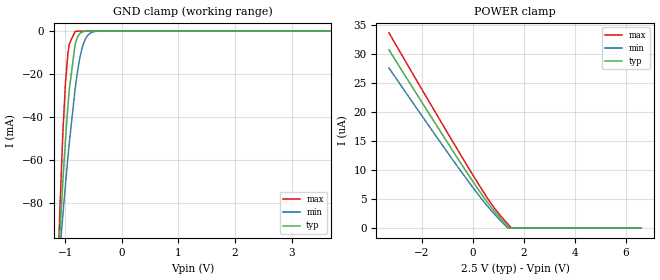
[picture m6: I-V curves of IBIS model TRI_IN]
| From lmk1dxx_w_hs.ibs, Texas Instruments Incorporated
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|   TRI_IN Model
[Model]   TRI_IN
Model_type   Input
Vinl = 0.75
Vinh = 1.75
|   typ   min   max
C_comp   1.93pF   1.8pF   2.08pF
[Voltage Range]   2.5   2.375   2.625
[Temperature Range]   45   150   -40
[Power Clamp Reference]   2.5   2.375   2.625
[GND Clamp Reference]   0   0   0
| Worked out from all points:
|   GND clamp passes 1 mA (typ) near -0.73 V on its own axis
[GND Clamp]
|   Voltage   I(typ)   I(min)   I(max)
-3.3V     -1.438A    -964.9mA   -2.518A
-1.104V   -99.63mA   -106.4mA   -92.28mA
-1.093V   -94.37mA   -102.8mA   -83.86mA
-1.046V   -72.35mA   -87.51mA   -50.86mA
-993.3mV  -50.29mA   -71.3mA    -23.68mA
-948.7mV  -34.08mA   -58.28mA   -9.883mA
-928mV    -27.51mA   -52.49mA   -6.1mA
-825mV    -6.468mA   -27.31mA   -175uA
-752.7mV  -1.574mA   -14.33mA   -15.03uA
-681.5mV  -227.7uA   -6.26mA    -9.726uA
-489.4mV  -7.798uA   -234uA     -8.143uA
6.6V      0A         0A         0A
[POWER Clamp]
|   Voltage   I(typ)   I(min)   I(max)
-3.3V     30.66uA    27.54uA    33.56uA
-1.312V   16.84uA    14.95uA    18.69uA
159.1mV   6.97uA     6.045uA    7.97uA
721.4mV   3.556uA    3.003uA    4.178uA
1.143V    1.396uA    1.012uA    1.813uA
1.373V    323.3nA    653.6pA    685.3nA
1.442V    4.024nA    0A         350.3nA
1.514V    0A         0A         1.632nA
6.6V      0A         0A         0A
